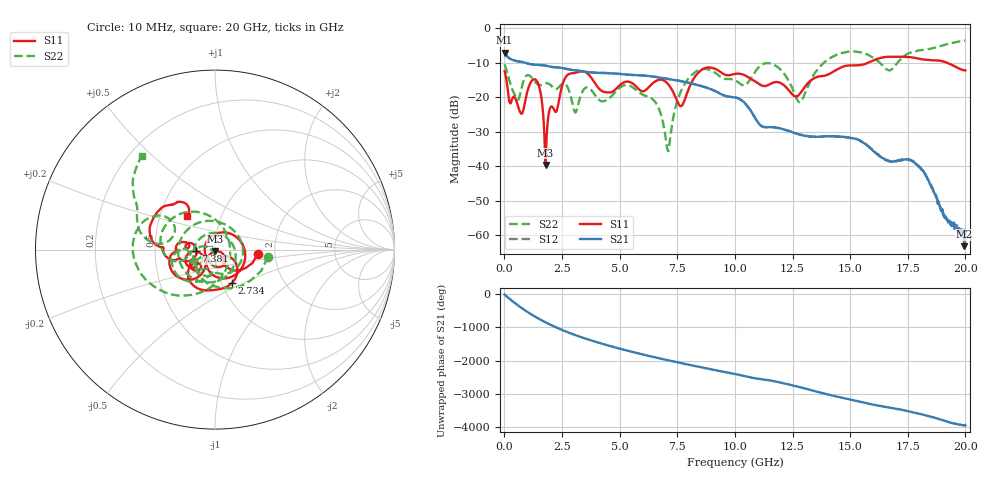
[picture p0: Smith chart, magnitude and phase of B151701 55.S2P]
!  2-Port S-parameters saved by WinCal
! VAR MeasName=S-Parameters (CALIBRATED_DATA) read from VNA (N5244A)
! VAR MeasDate=2015-12-24 19:16:22
! VAR NAME=B151701 55
! VAR FILENAME=B151701 55.S2P
! VAR DATE=2015-12-24 19:16:22
! VAR PHYS_PORTS=1,3
# Hz S DB R 50
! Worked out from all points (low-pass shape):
!   801 points, 10 MHz to 20 GHz, reference 50 ohm
!   highest |S21| = -7.13 dB at 10 MHz (marker M1); lowest = -63.2 dB at 19.95 GHz (marker M2)
!   |S21| within 3 dB of the highest: start of sweep to 942.3 MHz
!   lowest |S11| = -39.7 dB at 1.784 GHz (marker M3), VSWR 1.02, Z = 50.2 - j1.01 ohm
!   |S11| at or under -10 dB: start of sweep to 15.79 GHz; 19.19 GHz to end of sweep
!   |S22| runs from -35.7 to -3.6 dB; largest |S21 - S12| = 0.00095
!   S11 on the Smith chart (normalised r, x): 10 MHz: 1.62, -0.09; 2.734 GHz: 1.12, -0.43; 7.381 GHz: 0.81, -0.02; 20 GHz: 0.69, +0.27
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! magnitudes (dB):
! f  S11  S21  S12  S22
! 10 MHz  -12.5  -7.1  -7.1  -10.5
! 709.6 MHz  -24.7  -9.7  -9.7  -18.4
! 1.409 GHz  -15.3  -10.6  -10.6  -16.2
! 1.784 GHz  -39.7  -10.9  -10.9  -16.0
! 2.734 GHz  -13.6  -11.9  -11.9  -17.1
! 3.083 GHz  -12.9  -12.2  -12.2  -24.5
! 3.358 GHz  -12.5  -12.5  -12.5  -18.8
! 4.433 GHz  -18.6  -13.0  -13.0  -20.9
! 5.357 GHz  -15.5  -13.5  -13.5  -16.5
! 6.682 GHz  -15.1  -14.3  -14.3  -23.0
! 7.081 GHz  -16.1  -14.7  -14.7  -35.4
! 7.381 GHz  -19.4  -15.0  -15.0  -24.1
! 8.381 GHz  -13.1  -16.5  -16.5  -12.4
! 10.01 GHz  -13.3  -20.1  -20.1  -15.1
! 11.58 GHz  -16.0  -28.7  -28.6  -10.3
! 12.8 GHz  -19.2  -30.8  -30.8  -21.4
! 13.35 GHz  -14.9  -31.4  -31.4  -14.3
! 14.98 GHz  -10.8  -31.8  -31.8  -6.8
! 16.68 GHz  -8.3  -38.6  -38.5  -12.3
! 17.95 GHz  -8.8  -40.0  -39.8  -6.5
! 19.95 GHz  -12.2  -63.2  -57.8  -3.6
! 20 GHz  -12.3  -59.5  -59.6  -3.6
